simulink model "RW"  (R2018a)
settings: Solver=ode5  StartTime=0.0  StopTime=800  FixedStep=0.002  MaxStep=0.002  RelTol=1e-3  EnableMultiTasking=on
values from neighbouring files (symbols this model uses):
  Iw = 0.08    [run.m]
  Tmax = 0.05    [run.m]

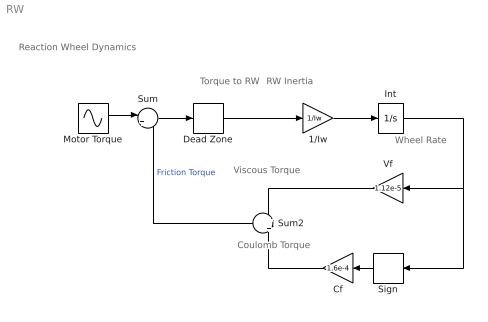
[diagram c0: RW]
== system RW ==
  note: Reaction Wheel Dynamics
  note: Torque to RW
  note: Wheel Rate
  note: RW Inertia
  note: Viscous Torque
  note: Coulomb Torque
  1/Iw : Gain  Gain=1/Iw
  Cf : Gain  Gain=1.6e-4
  Dead Zone : DeadZone  LowerValue=-1.6e-4  UpperValue=1.6e-4
  Int : Integrator
  Motor Torque : Sin  Amplitude=Tmax  Frequency=0.01  SampleTime=0
  Sign : Signum
  Sum : Sum  Inputs=|+-
  Sum2 : Sum  Inputs=+|+
  Vf : Gain  Gain=1.12e-5
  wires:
  Sum/1 -> Dead Zone/1
  Int/1 -> Sign/1, Vf/1
  Vf/1 -> Sum2/1
  Sign/1 -> Cf/1
  Dead Zone/1 -> 1/Iw/1
  Sum2/1 -> Sum/2  "Friction Torque"
  Motor Torque/1 -> Sum/1
  Cf/1 -> Sum2/2
  1/Iw/1 -> Int/1
